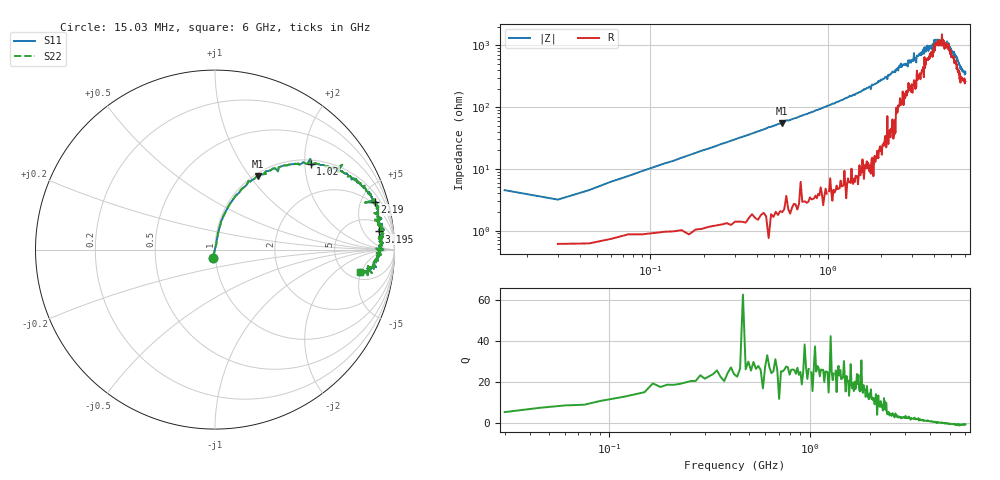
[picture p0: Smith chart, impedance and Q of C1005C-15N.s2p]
!	Network	Analyzer	HP8753E.07.74:	Oct	30	2002	Serial	No.	JP38451487
!	Hewlett-Packard
!	7	Sep	2009	8:46:56
!	Frequency	S11	S21	S12	S22
#	HZ	S	RI	R	50
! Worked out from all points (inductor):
!   400 points, 15.03 MHz to 6 GHz, reference 50 ohm
!   read as one part in series: L = 16.1 nH near 45.03 MHz
!   highest Q = 27.2 at 555 MHz (marker M1), where L = 15.8 nH
!   self-resonance near 4.328 GHz
!   S11 on the Smith chart (normalised r, x): 15.03 MHz: 0.97, -0.09; 1.02 GHz: 1.09, +2.14; 2.19 GHz: 1.69, +6.42; 3.195 GHz: 9, +11; 6 GHz: 6.25, -4.79
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1.502992e7  -0.0121 -0.0444  1.01 0.0444  1.01 0.0444  -0.0121 -0.0444
3.002985e7  0.00701 0.0308  0.993 -0.0308  0.993 -0.0308  0.00701 0.0308
9.002955e7  0.0166 0.0896  0.983 -0.0896  0.983 -0.0896  0.0166 0.0896
1.95029e8  0.0467 0.186  0.953 -0.186  0.953 -0.186  0.0467 0.186
5.550272e8  0.241 0.41  0.759 -0.41  0.759 -0.41  0.241 0.41
1.020025e9  0.533 0.479  0.467 -0.479  0.467 -0.479  0.533 0.479
2.01002e9  0.864 0.305  0.136 -0.305  0.136 -0.305  0.864 0.305
2.190019e9  0.889 0.265  0.111 -0.265  0.111 -0.265  0.889 0.265
3.015015e9  0.931 0.144  0.0692 -0.144  0.0692 -0.144  0.931 0.144
3.075015e9  0.941 0.111  0.059 -0.111  0.059 -0.111  0.941 0.111
3.165014e9  0.908 0.147  0.0924 -0.147  0.0924 -0.147  0.908 0.147
3.195014e9  0.912 0.101  0.0879 -0.101  0.0879 -0.101  0.912 0.101
3.91501e9  0.912 0.063  0.0882 -0.063  0.0882 -0.063  0.912 0.063
4.00501e9  0.934 0.0367  0.0663 -0.0367  0.0663 -0.0367  0.934 0.0367
4.03501e9  0.916 0.045  0.0842 -0.045  0.0842 -0.045  0.916 0.045
4.09501e9  0.934 0.0363  0.0656 -0.0363  0.0656 -0.0363  0.934 0.0363
4.365008e9  0.914 0.0214  0.086 -0.0214  0.086 -0.0214  0.914 0.0214
4.425008e9  0.938 -0.000427  0.0624 0.000427  0.0624 0.000427  0.938 -0.000427
4.455008e9  0.909 0.00568  0.0912 -0.00568  0.0912 -0.00568  0.909 0.00568
4.725006e9  0.925 -0.0281  0.0747 0.0281  0.0747 0.0281  0.925 -0.0281
5.010005e9  0.901 -0.0496  0.0989 0.0496  0.0989 0.0496  0.901 -0.0496
6e9  0.808 -0.127  0.192 0.127  0.192 0.127  0.808 -0.127
